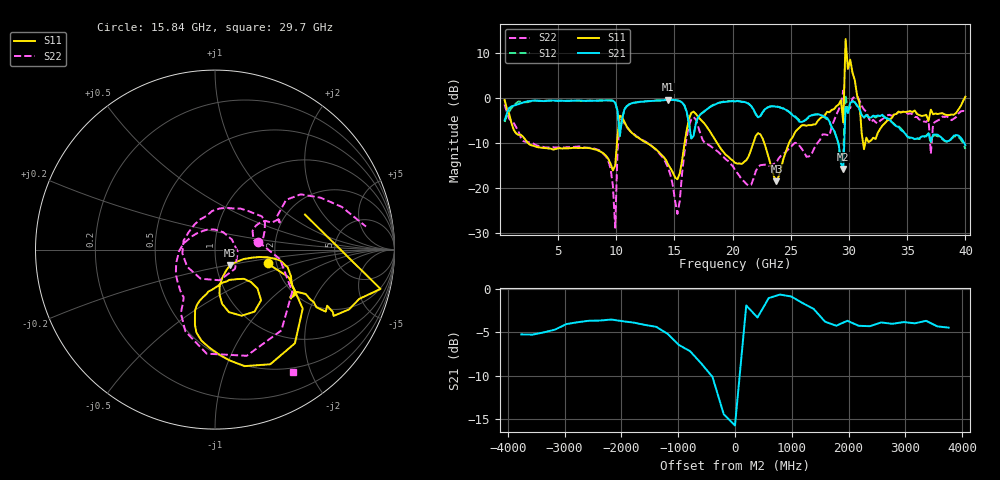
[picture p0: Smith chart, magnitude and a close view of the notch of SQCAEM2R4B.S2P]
! Network Analyzer HP8722ES.07.66: Jul 25, 2000 Serial No. US39175408
! 26 Oct 2004  13:13:04
! Frequency  S11  S21  S12  S22
# HZ  S  DB R  50
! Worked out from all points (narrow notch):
!   201 points, 400 MHz to 40 GHz, reference 50 ohm
!   highest |S21| = -0.34 dB at 14.46 GHz (marker M1); lowest = -15.7 dB at 29.51 GHz (marker M2)
!   notch at M2: 13.7 dB deep, 658 MHz wide at half that depth
!   lowest |S11| = -18.4 dB at 23.76 GHz (marker M3), VSWR 1.27, Z = 58.2 - j10.1 ohm
!   |S11| at or under -10 dB: 2.439 GHz to 10.06 GHz (7.617 GHz wide, 122 % of centre); 12.66 GHz to 15.87 GHz (3.206 GHz wide, 22.5 % of centre); 18.68 GHz to 21.77 GHz (3.09 GHz wide, 15.3 % of centre)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
!   |S22| runs from -28.7 to 1.7 dB; largest |S21 - S12| = 0.44
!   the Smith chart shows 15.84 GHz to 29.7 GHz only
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4e8  -0.39 -34.3  -4.88 57.3  -5.26 62.6  -1.39 -25.9
1.588e9  -8.15 -78.6  -1.31 16.6  -0.74 16.6  -7.37 -69.0
7.132e9  -11.05 -93.5  -0.57 -16.6  -0.59 -16.9  -10.90 -120.8
9.904e9  -14.96 -34.9  -0.96 -43.2  -0.94 -43.5  -28.71 86.0
1.03e10  -3.89 -48.0  -8.29 -36.8  -8.42 -34.1  -5.03 -46.4
1.3666e10  -11.98 -101.2  -0.52 -35.2  -0.47 -35.3  -12.18 -146.1
1.4458e10  -14.75 -94.6  -0.34 -41.2  -0.38 -41.4  -15.45 -159.5
1.525e10  -17.98 -55.1  -0.50 -51.3  -0.48 -51.2  -25.66 122.3
1.624e10  -4.60 -33.9  -5.50 -76.2  -5.58 -76.0  -6.19 -28.6
2.02e10  -14.34 -80.9  -0.74 -53.1  -0.65 -52.6  -15.88 160.3
2.3764e10  -18.41 -45.5  -1.89 -68.6  -1.82 -68.4  -14.25 103.8
2.6932e10  -5.82 -29.9  -3.67 -71.2  -3.74 -71.4  -11.54 30.4
2.9506e10  -5.39 21.2  -15.71 -162.8  -11.98 -129.6  1.73 29.2
2.9704e10  13.12 -46.1  -1.92 -55.0  0.71 -34.0  -1.83 -57.6
2.9902e10  6.50 -53.1  -3.30 -28.7  -3.34 -27.7  -2.23 4.7
3.01e10  8.56 -69.7  -1.06 -35.6  -1.07 -34.9  -2.22 4.2
3.0496e10  4.01 -84.9  -0.89 -62.1  -0.90 -60.1  0.34 -28.6
3.0694e10  0.58 79.0  -1.63 -75.2  -1.69 -73.1  0.47 138.7
3.1288e10  -11.31 83.9  -4.25 -76.9  -4.33 -76.6  -2.51 126.0
3.1486e10  -8.75 -68.4  -3.67 -72.7  -3.79 -72.8  -3.04 -54.1
3.3466e10  -4.75 -8.9  -4.68 -83.0  -4.86 -83.7  -3.68 -37.6
4e10  0.35 -29.8  -10.42 -112.7  -11.27 -110.8  -2.84 -36.8
